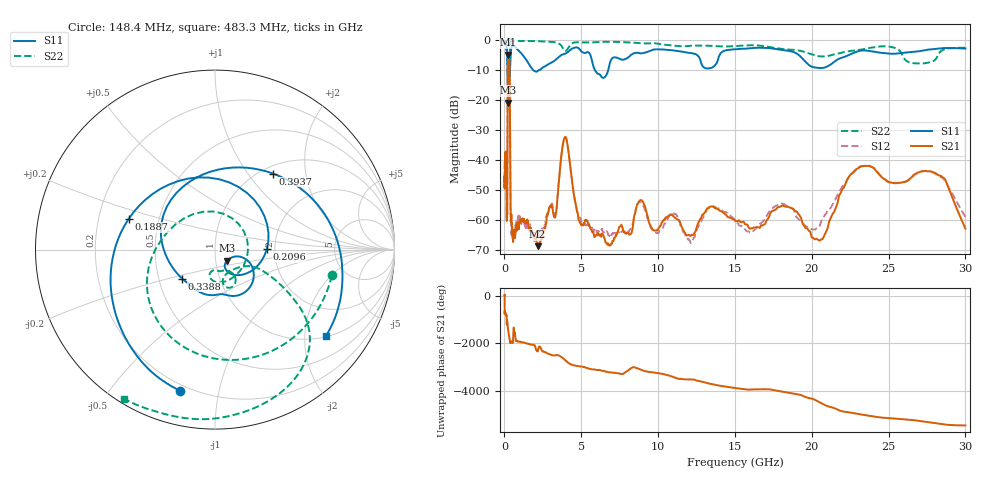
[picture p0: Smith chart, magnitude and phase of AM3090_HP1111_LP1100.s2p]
! Date/Time: Thu, Feb 28, 2019 2:10 PM
! Network Analyzer: Agilent Technologies E8364B Rev: A.07.50.67
! Sweep from 0.010 to 30.000 GHz, 1601 Points, Sweep Type: LOG
! Power Supply: 5.023 V, 0.002 A
# Hz S DB R 50
!freq MagS11 AngS11 MagS21 AngS21 MagS12 AngS12 MagS22 AngS22
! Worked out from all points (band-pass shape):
!   1601 points, 10 MHz to 30 GHz, reference 50 ohm
!   highest |S21| = -4.85 dB at 259.9 MHz (marker M1); lowest = -68.9 dB at 2.158 GHz (marker M2)
!   |S21| within 3 dB of the highest: 219.9 MHz to 327.3 MHz (107.4 MHz wide, 39.3 % of centre)
!   lowest |S11| = -20.9 dB at 243.5 MHz (marker M3), VSWR 1.20, Z = 56.7 - j6.97 ohm
!   |S11| at or under -10 dB: 207 MHz to 357.2 MHz (150.2 MHz wide, 53.2 % of centre); 1.865 GHz to 2.252 GHz (386.3 MHz wide, 18.8 % of centre); 5.886 GHz to 6.755 GHz (869.2 MHz wide, 13.8 % of centre)
!   |S22| runs from -18.8 to -0.1 dB; largest |S21 - S12| = 0.01
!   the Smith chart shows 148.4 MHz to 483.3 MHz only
!   S11 on the Smith chart (normalised r, x): 148.4 MHz: 0.17, -0.77; 188.7 MHz: 0.33, +0.15; 209.6 MHz: 1.81, +0.02; 338.8 MHz: 0.66, -0.23; 393.7 MHz: 1.13, +1.33; 483.3 MHz: 1.03, -2.55
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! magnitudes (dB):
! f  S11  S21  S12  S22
! 10 MHz  -0.3  -47.3  -40.6  -0.6
! 38.04 MHz  -0.2  -40.9  -40.5  -1.2
! 96.49 MHz  -0.8  -38.4  -38.7  -2.8
! 144.7 MHz  -1.7  -57.7  -55.6  -3.5
! 148.4 MHz  -1.8  -59.7  -57.7  -3.5
! 188.7 MHz  -5.8  -49.5  -49.6  -7.4
! 209.6 MHz  -10.8  -13.4  -13.4  -14.7
! 243.5 MHz  -20.9  -5.2  -5.1  -18.1
! 259.9 MHz  -15.9  -4.9  -4.8  -17.2
! 338.8 MHz  -12.3  -10.8  -10.8  -8.0
! 393.7 MHz  -5.5  -53.0  -53.1  -0.8
! 483.3 MHz  -2.1  -63.8  -64.1  -0.2
! 550.5 MHz  -2.0  -66.4  -67.3  -0.2
! 2.084 GHz  -10.6  -67.1  -64.3  -0.4
! 2.158 GHz  -10.4  -68.9  -65.5  -0.4
! 3.302 GHz  -6.7  -59.2  -58.5  -0.8
! 3.934 GHz  -4.6  -32.4  -32.4  -3.6
! 4.977 GHz  -3.6  -61.7  -59.8  -0.7
! 7.926 GHz  -6.2  -64.7  -64.0  -0.7
! 20.31 GHz  -9.2  -66.3  -62.9  -5.2
! 23.48 GHz  -3.5  -42.0  -42.0  -2.9
! 30 GHz  -2.8  -63.0  -59.1  -2.6
